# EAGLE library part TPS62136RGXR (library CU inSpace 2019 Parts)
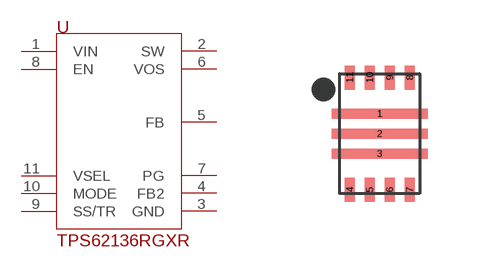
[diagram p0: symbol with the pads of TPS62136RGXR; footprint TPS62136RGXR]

Designator prefix U

## TPS62136RGXR  [TPS62136RGXR]
1  VIN
2  SW
3  GND
4  FB2
5  FB
6  VOS
7  PG
8  EN
9  SS/TR
10  MODE
11  VSEL

## Footprint TPS62136RGXR (pad centres in mm)
smd 2.4 x 0.25: 1 0,0.5; 2 0,0; 3 0,-0.5
smd 0.25 x 0.6: 4 -0.75,-1.4; 5 -0.25,-1.4; 6 0.25,-1.4; 7 0.75,-1.4; 8 0.75,1.4; 9 0.25,1.4; 10 -0.25,1.4; 11 -0.75,1.4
